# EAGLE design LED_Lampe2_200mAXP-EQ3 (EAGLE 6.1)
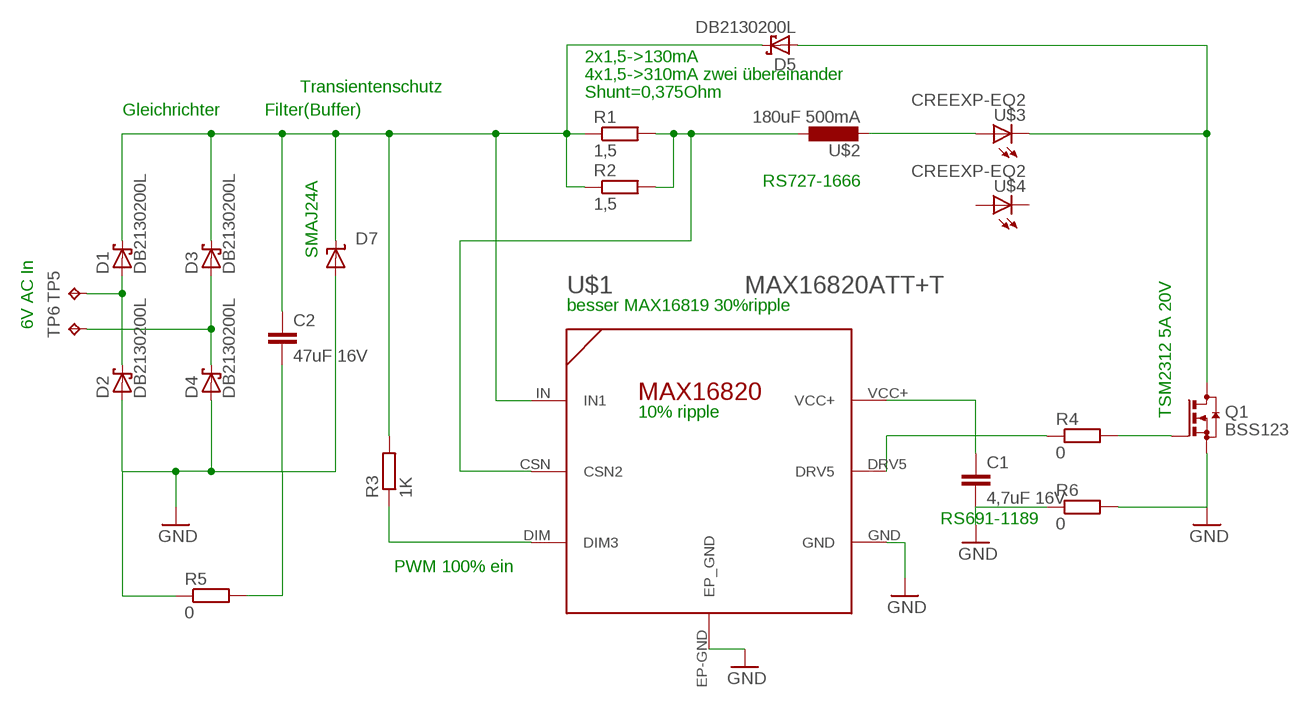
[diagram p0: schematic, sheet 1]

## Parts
C1  4,7uF 16V  C-EUC1206  [C1206]
C2  47uF 16V  C-EUC1812K  [C1812K]
D1  DB2130200L  [SMINI2]
D2  DB2130200L  [SMINI2]
D3  DB2130200L  [SMINI2]
D4  DB2130200L  [SMINI2]
D5  DB2130200L  [SMINI2]
D7  SUPPRESSOR-SMBJ  [SMBJ]
Q1  BSS123  [SOT23]
R1  1,5  R-EU_R0805  [R0805]
R2  1,5  R-EU_R0805  [R0805]
R3  1K  R-EU_R1206  [R1206]
R4  0  R-EU_R1206  [R1206]
R5  0  R-EU_R1206  [R1206]
R6  0  R-EU_R1206  [R1206]
TP5  TPTP20SQ  [TP20SQ]
TP6  TPTP20SQ  [TP20SQ]
U$1  MAX16820ATT+T  [TDFN6]
U$2  180uF 500mA  L-EU-SMD  [L8X8MM]
U$3  CREEXP-EQ2  [CREE_XPEQ2]
U$4  CREEXP-EQ2  [CREE_XPEQ2]

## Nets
GND: C1.2 C2.2 D2.A2(A) D4.A2(A) D7.A Q1.2(S) R5.1 R5.2 R6.1 R6.2 U$1.EP-GND(EP_GND) U$1.GND
N$1: U$2.P$2 U$3.1A(A)
N$3: Q1.1(G) R4.2
N$4: R4.1 U$1.DRV5
N$5: D5.A2(A) Q1.3(D) U$3.2K(C)
N$6: R1.2 R2.2 U$1.CSN(CSN2) U$2.P$1
N$7: C2.1 D1.K1(C) D3.K1(C) D5.K1(C) D7.C R1.1 R2.1 R3.2 U$1.IN(IN1)
N$9: R3.1 U$1.DIM(DIM3)
N$11: D1.A2(A) D2.K1(C) TP5.TP
N$12: D3.A2(A) D4.K1(C) TP6.TP
VCC+: C1.1 U$1.VCC+
Unconnected: U$4.1A(A) U$4.2K(C)

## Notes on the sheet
- 2x1,5->130mA
- Transientenschutz | 4x1,5->310mA zwei übereinander
- Shunt=0,375Ohm
- Gleichrichter | Filter(Buffer)
- RS727-1666
- SMAJ24A
- besser MAX16819 30%ripple
- 6V AC In
- 10% ripple | TSM2312 5A 20V
- RS691-1189
- PWM 100% ein

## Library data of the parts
C1 C2 = rcl:C-EU: CAPACITOR, European symbol
D1-D5 = diode_modif:DB2130200L
D7 = Diode_mod:SUPPRESSOR-: Suppressor diode
Q1 = transistor-small-signal:BSS123: N-CHANNEL MOS FET
R1-R6 = rcl:R-EU_: RESISTOR, European symbol
TP5 TP6 = testpad:TP: Test pad
U$1 = maxim_mod:MAX16820ATT+T
U$2 = rcl:L-EU-SMD: round 8mm diameter SMD Inductor SDR0805 Series
U$3 U$4 = led:CREEXP-EQ2

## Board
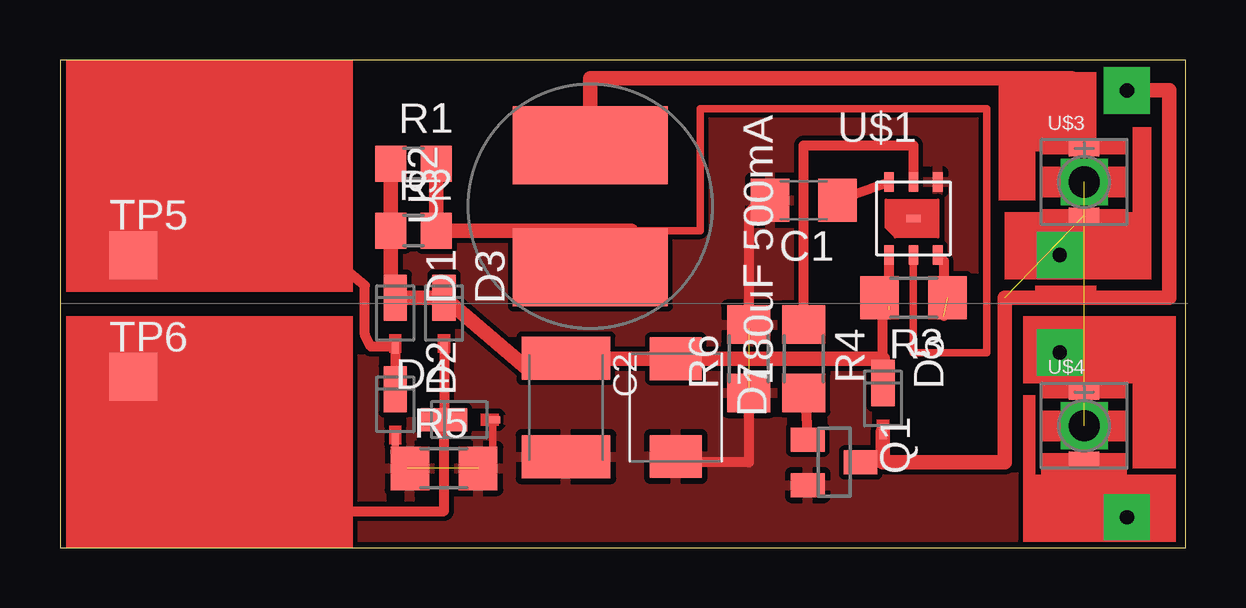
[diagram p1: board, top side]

Size 46.91 x 20.31 mm. Coordinates in mm from the lower left corner, seen from the top.
Outline: 0,0 46.91,0 46.91,20.31 0,20.31 0,0
Copper layers (1*16): Top 0.035mm / dielectric 1.5mm / Bottom 0.035mm
Design rules: minimum track width 10mil, minimum drill 24mil, track to track 8mil, track to pad 8mil, pad to pad 8mil, via to via 8mil, smd to smd 8mil, copper to edge 10mil, drill to drill 8mil, minimum pad ring 10mil, minimum via ring 8mil, stop-mask expansion 4mil, vias tented up to drill 0mil, thermal gap 10mil

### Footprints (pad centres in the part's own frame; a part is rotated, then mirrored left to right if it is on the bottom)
C1206 = smd 1.6 x 1.8: 1 -1.4,0; 2 1.4,0
C1812K = smd 1.8 x 3.7: 1 -2.05,0; 2 2.05,0
SMINI2 = smd 0.305 x 0.61: A2 0,0.762 | smd 0.965 x 1.93: K1 0,-1.27
SMBJ = smd 1.78 x 2.16: A 2.04,0; C -2.03,0
SOT23 = smd 1 x 1.4: 1 -0.95,-1.1; 2 0.95,-1.1; 3 0,1.1
R0805 = smd 1.3 x 1.5: 1 -0.95,0; 2 0.95,0
R1206 = smd 1.6 x 1.803: 1 -1.422,0; 2 1.422,0
TP20SQ = smd 2 x 2: TP 0,0
TDFN6 = smd 0.406 x 0.813: CSN 0,-1.524; DIM 1.016,-1.524; DRV5 0,1.524; GND 1.016,1.524; IN -1.016,-1.524; VCC+ -1.016,1.524 | smd 0.61 x 0.305: EP-GND 0,0
L8X8MM = smd 6.452 x 3.251: P$1 0,2.54; P$2 0,-2.54
CREE_XPEQ2 = smd 1.27 x 0.635: 1A 0,1.397; 2K 0,-1.397

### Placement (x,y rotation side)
C1  30.99,14.48 180 top
C2  21.08,5.84 270 top
D1  13.97,9.14 180 top
D2  13.97,5.33 180 top
D3  16,9.14 180 top
D4  17.27,5.33 270 top
D5  34.29,5.59 180 top
D7  25.65,5.84 270 top
Q1  32.26,3.56 270 top
R1  14.73,16 0 top
R2  14.73,13.21 0 top
R3  35.56,10.41 180 top
R4  30.99,7.87 270 top
R5  16,3.3 0 top
R6  28.7,7.87 90 top
TP5  3.05,12.19 0 top
TP6  3.05,7.11 0 top
U$1  35.56,13.72 0 top
U$2  22.1,14.22 180 top
U$3  42.67,15.24 0 top
U$4  42.67,5.08 0 top

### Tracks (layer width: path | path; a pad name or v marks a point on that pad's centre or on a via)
GND  (3 unrouted)
  Top 0.305: D2.A2 13.97,3.56 14.48,3.3 | R5.2 18.03,3.56 D4.A2
  Top 0.406: C1.2 29.21,14.48 28.7,13.97 28.7,9.14 | R6.1 28.7,3.56 25.9,3.56 D7.A
  pour Top: -0.51,20.32 47.24,20.57 47.24,-0.25 -0.51,-0.51
N$1
  Top 0.61: U$2.P$2 22.1,19.56 42.16,19.56 42.67,19.05 U$3.1A 42.67,16.51
N$2  (via drill 1.3 pad 1.78)  (1 unrouted)
  other vias: 42.67,15.24 42.67,5.08
N$3
  Top 0.406: R4.2 31.03,6.42 Q1.1
N$4
  Top 0.406: R4.1 30.99,16.76 35.56,16.76 U$1.DRV5
N$5  (1 unrouted)
  Top 0.406: Q1.3 34.29,3.56
  Top 0.61: 44.45,19.05 46.23,19.05 46.23,10.41 39.37,10.41 39.37,3.56 34.29,3.56 D5.A2
N$6
  Top 0.305: 23.81,13.21 26.67,13.21 26.67,18.29 38.61,18.29 38.61,8.13 35.56,8.13 U$1.CSN
  Top 0.406: U$2.P$1 22.1,13.21
  Top 0.61: R1.2 R2.2 22.1,13.21 23.81,13.21
N$7  (1 unrouted)
  Top 0.406: D1.K1 13.78,10.6 | R3.2 34.54,10.06 U$1.IN | 21.46,7.87 C2.1 | 34.29,7.87 34.29,10.16 34.54,9.91 | 34.29,7.87 | 34.29,7.87 D5.K1
  Top 0.61: D1.K1 D3.K1 19.43,7.5 C2.1 | 13.78,10.6 R2.1 R1.1 | 21.46,7.87 D7.C 34.29,7.87
N$8  (via drill 0.6 pad 1.93)
  other vias: 41.66,12.19
N$9  (1 unrouted)
  Top 0.406: U$1.DIM 36.83,11.94 36.83,9.65
N$10  (via drill 0.6 pad 1.93)
  other vias: 44.45,19.05
N$11
  Top 0.406: D2.K1 D1.A2 12.95,8.38 12.7,8.89 12.7,10.92 11.18,12.19 TP5.TP
N$12
  Top 0.406: D3.A2 D4.K1 16,1.52 10.41,1.52 10.41,7.11 TP6.TP
N$13  (via drill 0.6 pad 1.93)
  other vias: 41.66,8.13
N$14  (via drill 0.6 pad 1.93)
  other vias: 44.45,1.27
VCC+
  Top 0.406: C1.1 U$1.VCC+
(copper drawn outside any net)
  shapes: Top area x12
